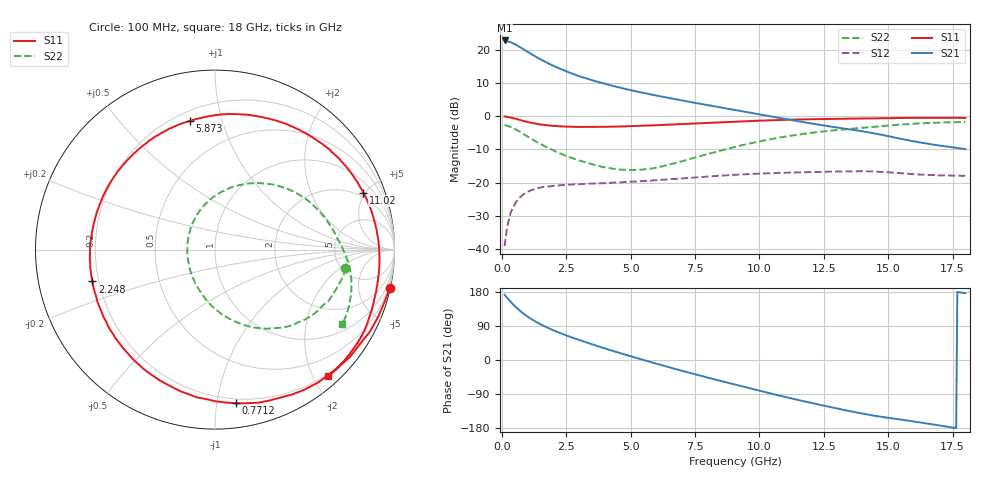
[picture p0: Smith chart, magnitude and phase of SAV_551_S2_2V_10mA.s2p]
! Data provided by Modelithics, Inc.  Tampa, Florida USA, June 2008
!Model SAV-551+
!VAR V_out= 2
!VAR I_out= 10
!VAR V_in= 0.3062
!VAR I_in= 0.8550
!BEGIN ACDATA
# GHZ S MA R 50
! Scattering Parameters
!% F n11x n11y n21x n21y n12x n12y n22x n22y
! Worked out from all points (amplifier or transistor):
!   401 points, 100 MHz to 18 GHz, reference 50 ohm
!   highest |S21| = 22.9 dB at 100 MHz (marker M1)
!   |S21| within 3 dB of that: start of sweep to 902.1 MHz
!   unconditionally stable (mu >= 1): 4.914 GHz to 10.6 GHz
!   at 3.054 GHz: K = 0.70, MSG = 16.2 dB, |S12| = -20.5 dB
!   at 9.05 GHz: K = 1.09, MAG = 8.0 dB, |S12| = -17.7 dB
!   at 18 GHz: K = 0.88, MSG = 4.0 dB, |S12| = -18.0 dB
!   lowest NFmin = 0.09 dB at 500 MHz
!   S11 on the Smith chart (normalised r, x): 100 MHz: 0.10, -9.26; 771.2 MHz: 0.17, -1.13; 2.248 GHz: 0.18, -0.12; 5.873 GHz: 0.26, +0.79; 11.02 GHz: 1.68, +4.87; 18 GHz: 0.17, -2.22
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0.1  0.9977 -12.3  13.96 172.3  0.01097 82.3  0.7335 -8.1
0.1895  0.9829 -22.5  13.56 164.7  0.02026 76.4  0.7218 -14.1
0.279  0.9643 -32.7  13.26 157.4  0.02842 68.9  0.7027 -20.8
0.3685  0.9488 -43.4  12.95 150.9  0.03743 65.8  0.6762 -27.4
0.458  0.9361 -52.6  12.43 145.0  0.04401 60.1  0.6574 -33.0
0.59225  0.9006 -66.3  11.66 136.1  0.05376 53.4  0.6147 -41.3
0.77125  0.8641 -82.2  10.62 125.8  0.06341 45.3  0.5606 -51.1
0.9055  0.835 -93.1  9.868 118.8  0.06924 40.5  0.5214 -57.6
1.0845  0.8043 -106.5  8.945 110.3  0.07517 34.0  0.4718 -65.6
1.39775  0.7635 -126.2  7.604 97.8  0.0823 25.5  0.3992 -77.0
1.8005  0.7263 -146.8  6.283 84.2  0.08725 17.5  0.3324 -89.5
2.248  0.7055 -165.4  5.229 71.4  0.09108 10.5  0.2765 -101.6
3.09825  0.69 166.2  3.924 50.3  0.09493 1.0  0.2096 -123.3
4.396  0.6987 132.3  2.819 22.1  0.09996 -9.7  0.1606 -160.2
5.87275  0.7302 100.9  2.103 -7.3  0.1079 -19.6  0.1649 152.6
6.0965  0.738 96.7  2.024 -11.6  0.1095 -21.4  0.1724 145.4
7.439  0.7777 73.1  1.612 -36.5  0.1187 -31.6  0.2344 110.8
9.05  0.8286 48.4  1.243 -64.9  0.1308 -45.4  0.3448 78.3
11.019  0.8848 20.9  0.9087 -97.8  0.1406 -65.8  0.4948 46.2
12.04825  0.9047 8.1  0.7779 -113.7  0.1445 -77.0  0.5655 31.9
15.0465  0.9379 -23.3  0.4982 -153.0  0.1424 -107.2  0.728 -2.5
18  0.9439 -48.3  0.3192 176.3  0.1264 -132.3  0.8221 -30.4
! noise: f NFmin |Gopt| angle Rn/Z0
0.5  0.085  0.3861  26.58  0.092
0.7  0.12  0.3948  36.23  0.083
0.9  0.155  0.4034  45.77  0.075
1  0.172  0.4077  50.49  0.072
1.9  0.331  0.4455  91.76  0.049
2.4  0.418  0.4659  113.7  0.044
3  0.524  0.4897  139.1  0.044
3.9  0.682  0.5243  175.3  0.059
5  0.875  0.5645  -143.5  0.099
6  1.051  0.5992  -109  0.157
